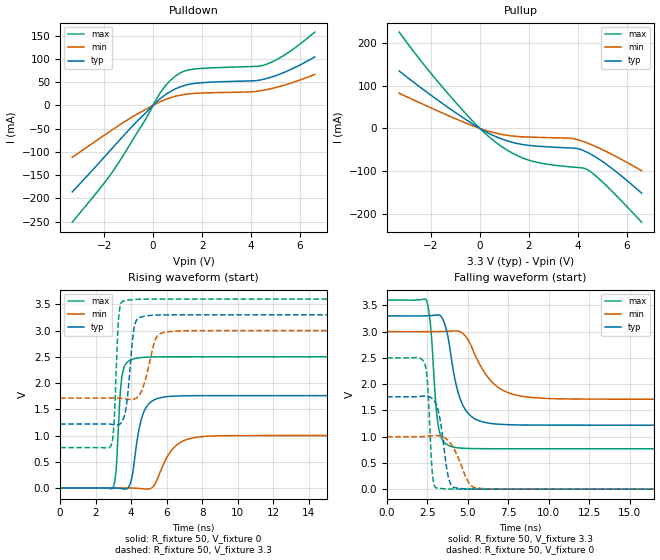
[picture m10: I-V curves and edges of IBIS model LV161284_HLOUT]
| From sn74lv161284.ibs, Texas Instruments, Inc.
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[Model]   LV161284_HLOUT
Model_type  Output
Vref =   0
Rref =   500
Cref =   50p
Vmeas =   1.4
| variable   typ   min   max
C_comp   4.18pF   2.71pF   5.56pF
| C_pullup   4.22pF   2.71pF   5.35pF
| C_pulldown   4.14pF   3.00pF   5.56pF
[Temperature Range]   40   100   -40
| Ambient temperature   25   85   -40
[Voltage range]   3.3   3   3.6
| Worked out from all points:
|   slope of the pulldown table from 0 to 0.495 V, typ, clamps not added: 21.9 ohm
|   slope of the pullup table from 0 to 0.495 V, typ, clamps not added: 32.9 ohm
|   rising waveform, R_fixture 50, V_fixture 0: 20-80 % time 552ps typ, 991ps min, 255ps max; typ from 0 V to 1.76 V
|   falling waveform, R_fixture 50, V_fixture 3.3: 20-80 % time 853ps typ, 1.55ns min, 396ps max; typ from 3.3 V to 1.22 V
|   rising waveform, R_fixture 50, V_fixture 3.3: 20-80 % time 340ps typ, 564ps min, 200ps max; typ from 1.22 V to 3.3 V
|   falling waveform, R_fixture 50, V_fixture 0: 20-80 % time 484ps typ, 832ps min, 247ps max; typ from 1.76 V to 0 V
[Pulldown]
| LV161284_HLOUT
|   Voltage   I(typ)   I(min)   I(max)
-3.3V     -186.1mA   -111.8mA   -251.2mA
-1.685V   -93.22mA   -53.35mA   -145mA
-375mV    -20.06mA   -11mA      -35.79mA
275mV     13.64mA    7.441mA    25.46mA
565mV     25.07mA    13.75mA    45.69mA
880mV     34.49mA    18.95mA    61.51mA
1.23V     41.8mA     22.92mA    72.59mA
1.62V     46.54mA    25.38mA    77.55mA
3.95V     52.36mA    28.8mA     83.24mA
4.555V    56.56mA    32.9mA     86.99mA
5.45V     72.99mA    44.81mA    111mA
6.6V      104mA      66.36mA    157.4mA
[Pullup]
| LV161284_HLOUT
|   Voltage   I(typ)   I(min)   I(max)
-3.3V     133.9mA    82.14mA    224.4mA
-2.27V    88.81mA    54.94mA    147.4mA
-1.18V    44.1mA     27.2mA     73mA
-170mV    5.902mA    3.555mA    9.673mA
595mV     -17.64mA   -10.14mA   -29.89mA
1.31V     -32.09mA   -17.38mA   -56.97mA
2.02V     -39.45mA   -20.04mA   -74.15mA
3.695V    -45.44mA   -22.81mA   -89.41mA
4.035V    -47.63mA   -26.96mA   -91.04mA
4.385V    -55.61mA   -33.93mA   -95.92mA
5.135V    -82.36mA   -53mA      -131.7mA
6.6V      -150.6mA   -98.47mA   -218.2mA
[Ramp]
| LV161284_HLOUT
| variable   typ   min   max
dV/dt_r   1.07/5.60E-10   0.61/9.96E-10   1.51/2.65E-10
dV/dt_f   1.26/8.60E-10   0.78/1.56E-09   1.71/4.09E-10
R_load = 50
[Rising Waveform]
| LV161284_HLOUT
R_fixture =   50
C_fixture =   0
L_fixture =   0
V_fixture =   0
V_fixture_min = 0
V_fixture_max = 0
|   Time   V(typ)   V(min)   V(max)
0s        104.2pV    215.6pV    40.77pV
2.955ns   1.066mV    1.502uV    -6.126mV
3.145ns   -148.3uV   154.1uV    315.5mV
3.52ns    -13.47mV   606.4uV    2.201V
3.99ns    132.1mV    -411.3uV   2.442V
4.535ns   1.26V      -10.54mV   2.484V
5.42ns    1.698V     127.6mV    2.498V
6.545ns   1.753V     814.6mV    2.5V
8.44ns    1.76V      989.4mV    2.501V
70ns      1.76V      999.8mV    2.501V
[Falling Waveform]
| LV161284_HLOUT
R_fixture =   50
C_fixture =   0
L_fixture =   0
V_fixture =   3.3
V_fixture_min = 3
V_fixture_max = 3.6
|   Time   V(typ)   V(min)   V(max)
0s        3.3V       3V         3.6V
2.425ns   3.301V     2.999V     3.603V
2.68ns    3.305V     2.999V     3.143V
3.215ns   3.317V     3.001V     1.129V
3.685ns   3.014V     3.006V     853.4mV
4.32ns    1.927V     3.013V     790.2mV
5.56ns    1.319V     2.475V     771.9mV
6.995ns   1.235V     1.912V     769.7mV
9.375ns   1.22V      1.736V     769.5mV
70ns      1.219V     1.714V     769.4mV
[Rising Waveform]
| LV161284_HLOUT
R_fixture =   50
C_fixture =   0
L_fixture =   0
V_fixture =   3.3
V_fixture_min = 3
V_fixture_max = 3.6
|   Time   V(typ)   V(min)   V(max)
0s        1.219V     1.714V     769.4mV
2.85ns    1.216V     1.714V     800.5mV
3.045ns   1.205V     1.715V     1.291V
3.33ns    1.211V     1.711V     3.365V
3.675ns   1.46V      1.698V     3.57V
3.935ns   2.273V     1.687V     3.585V
4.325ns   3.21V      1.723V     3.594V
5.425ns   3.295V     2.872V     3.599V
6.48ns    3.299V     2.99V      3.6V
70ns      3.3V       3V         3.6V
[Falling Waveform]
| LV161284_HLOUT
R_fixture =   50
C_fixture =   0
L_fixture =   0
V_fixture =   0
V_fixture_min = 0
V_fixture_max = 0
|   Time   V(typ)   V(min)   V(max)
0s        1.76V      999.8mV    2.501V
2.305ns   1.775V     1.004V     2.412V
2.5ns     1.77V      1.01V      2.025V
2.84ns    1.71V      1.02V      202.5mV
3.37ns    1.145V     1.006V     11.31mV
3.885ns   128.6mV    891.4mV    2.755mV
4.735ns   7.297mV    330mV      375.8uV
5.31ns    2.132mV    41.7mV     109.3uV
6.64ns    234.2uV    3.399mV    8.612uV
70ns      567pV      229.2pV    309.4pV
